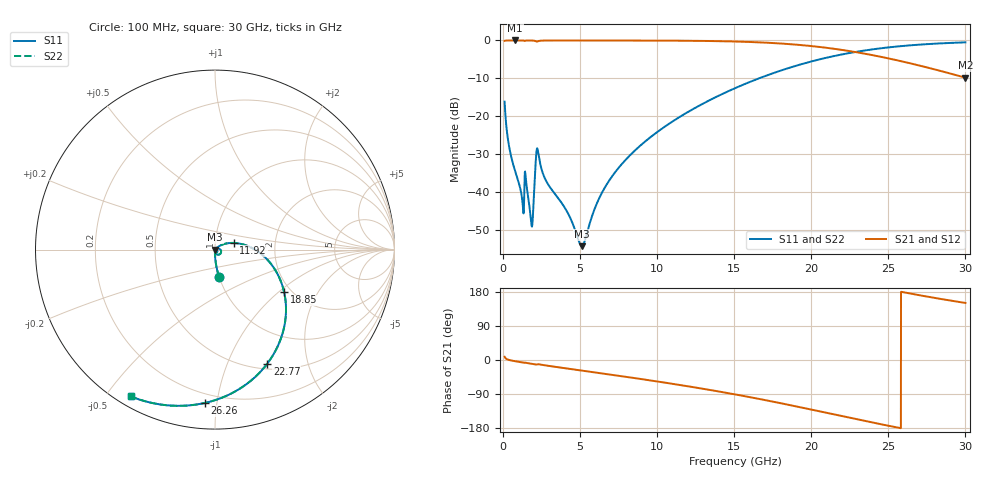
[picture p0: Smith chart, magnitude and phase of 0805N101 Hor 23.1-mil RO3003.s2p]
# GHz S MA R 50
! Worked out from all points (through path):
!   3201 points, 100 MHz to 30 GHz, reference 50 ohm
!   highest |S21| = -0.01 dB at 791.4 MHz (marker M1); lowest = -9.8 dB at 30 GHz (marker M2)
!   group delay of S21, straight-line fit = 20.1 ps
!   lowest |S11| = -54.3 dB at 5.108 GHz (marker M3), VSWR 1.00, Z = 50.2 - j0.0931 ohm
!   |S11| at or under -10 dB: start of sweep to 16.61 GHz
!   |S22| runs from -54.3 to -0.5 dB; largest |S21 - S12| = 0
!   S11 on the Smith chart (normalised r, x): 100 MHz: 1.00, -0.31; 11.92 GHz: 1.23, +0.09; 18.85 GHz: 1.83, -1.10; 22.77 GHz: 0.56, -1.40; 26.26 GHz: 0.14, -0.92; 30 GHz: 0.04, -0.58
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0.1  0.1558 -81.5  0.9876 8.4  0.9876 8.4  0.1558 -81.5
0.399  0.03903 -89.4  0.9988 0.0  0.9988 0.0  0.03903 -89.4
0.7914375  0.01863 -91.5  0.9992 -3.3  0.9992 -3.3  0.01863 -91.5
1.22125  0.008503 -87.9  0.9987 -6.2  0.9987 -6.2  0.008503 -87.9
1.529594  0.01187 -83.5  0.997 -7.8  0.997 -7.8  0.01187 -83.5
1.837938  0.003735 -51.2  0.9971 -10.0  0.9971 -10.0  0.003735 -51.2
1.950063  0.005461 11.4  0.9949 -10.8  0.9949 -10.8  0.005461 11.4
2.155625  0.03227 -5.7  0.9678 -12.0  0.9678 -12.0  0.03227 -5.7
2.277094  0.0336 -58.7  0.977 -11.1  0.977 -11.1  0.0336 -58.7
2.753625  0.01452 -91.6  0.9966 -14.3  0.9966 -14.3  0.01452 -91.6
5.089563  0.001929 -32.0  0.9979 -27.7  0.9979 -27.7  0.001929 -32.0
5.10825  0.001925 -28.8  0.9979 -27.8  0.9979 -27.8  0.001925 -28.8
6.930281  0.01459 43.3  0.9975 -38.2  0.9975 -38.2  0.01459 43.3
10.06978  0.06321 30.5  0.9949 -57.0  0.9949 -57.0  0.06321 30.5
11.91984  0.1113 19.5  0.9902 -68.9  0.9902 -68.9  0.1113 19.5
15.05  0.2341 -1.7  0.9677 -90.7  0.9677 -90.7  0.2341 -1.7
18.85291  0.4529 -31.7  0.8856 -121.0  0.8856 -121.0  0.4529 -31.7
20.03956  0.5301 -41.8  0.8415 -131.2  0.8415 -131.2  0.5301 -41.8
22.76794  0.6989 -65.4  0.7079 -154.8  0.7079 -154.8  0.6989 -65.4
25.01978  0.8099 -84.1  0.5786 -173.6  0.5786 -173.6  0.8099 -84.1
26.2625  0.8566 -93.8  0.5076 176.6  0.5076 176.6  0.8566 -93.8
30  0.9433 -119.9  0.3223 150.6  0.3223 150.6  0.9433 -119.9
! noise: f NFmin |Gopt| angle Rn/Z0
0.1  0.000347  0.8295  0.7091  0.0004287
3.417  0.006351  0.7054  18.74  0.004124
6.743  0.009116  0.6223  36.35  0.004093
10.06  0.0125  0.6045  52.89  0.004752
13.39  0.01631  0.6081  68.27  0.005421
16.7  0.02082  0.6254  82.45  0.006124
20.03  0.02654  0.6539  95.73  0.006922
23.35  0.03414  0.6922  108.4  0.007867
26.67  0.0449  0.7393  120.8  0.00899
30  0.06107  0.7921  133.4  0.01017
